FUNCTION "Gest Consensi 2ndCC" : VOID
TITLE =
VERSION : 0.1

BEGIN
NETWORK
TITLE =Condizioni di Sicurezza OK
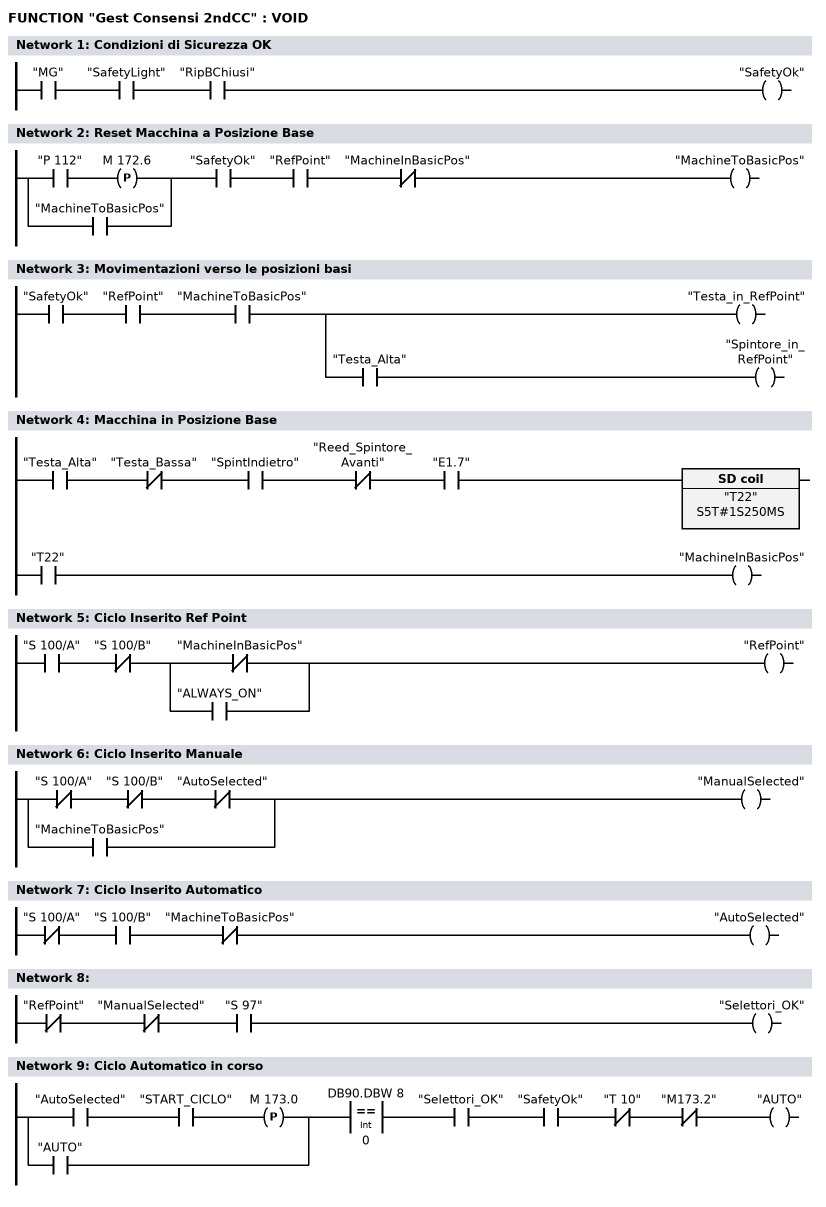
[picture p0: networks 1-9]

      U     "MG";
      U     "SafetyLight";
      U     "RipBChiusi";
      =     "SafetyOk";
NETWORK
TITLE =Reset Macchina a Posizione Base

      U(    ;
      U     "P 112";
      FP    M    172.6;
      O     "MachineToBasicPos";
      )     ;
      U     "SafetyOk";
      U     "RefPoint";
      UN    "MachineInBasicPos";
      =     "MachineToBasicPos";
NETWORK
TITLE =Movimentazioni verso le posizioni basi

      U     "SafetyOk";
      U     "RefPoint";
      U     "MachineToBasicPos";
      =     L      0.0;
      U     L      0.0;
      BLD   102;
      =     "Testa_in_RefPoint";
      U     L      0.0;
      U     "Testa_Alta";
      =     "Spintore_in_RefPoint";
NETWORK
TITLE =Macchina in Posizione Base

      U     "Testa_Alta";
      UN    "Testa_Bassa";
      U     "SpintIndietro";
      UN    "Reed_Spintore_Avanti";
      U     "E1.7";
      L     S5T#1S250MS;
      SE    "T22";
      NOP   0;
      NOP   0;
      NOP   0;
      U     "T22";
      =     "MachineInBasicPos";
NETWORK
TITLE =Ciclo Inserito Ref Point

      U     "S 100/A";
      UN    "S 100/B";
      U(    ;
      ON    "MachineInBasicPos";
      O     "ALWAYS_ON";
      )     ;
      =     "RefPoint";
NETWORK
TITLE =Ciclo Inserito Manuale

      UN    "S 100/A";
      UN    "S 100/B";
      UN    "AutoSelected";
      O     "MachineToBasicPos";
      =     "ManualSelected";
NETWORK
TITLE =Ciclo Inserito Automatico

      UN    "S 100/A";
      U     "S 100/B";
      UN    "MachineToBasicPos";
      =     "AutoSelected";
NETWORK
TITLE =

      UN    "RefPoint";
      UN    "ManualSelected";
      U     "S 97";
      =     "Selettori_OK";
NETWORK
TITLE =Ciclo Automatico in corso

      U(    ;
      U     "AutoSelected";
      U     "START_CICLO";
      FP    M    173.0;
      O     "AUTO";
      )     ;
      U(    ;
      L     DB90.DBW    8;
      L     0;
      ==I   ;
      )     ;
      U     "Selettori_OK";
      U     "SafetyOk";
      UN    "T 10";
      UN    "M173.2";
      =     "AUTO";
NETWORK
TITLE =Funzioni di toggle sul pulsante di start

      U(    ;
      U     "AUTO";
      UN    "START_CICLO";
      L     S5T#300MS;
      SE    "T40";
      NOP   0;
      NOP   0;
      NOP   0;
      U     "T40";
      )     ;
      S     "M173.1";
      U(    ;
      ON    "AUTO";
      ON    "AutoSelected";
      )     ;
      R     "M173.1";
      NOP   0;
NETWORK
TITLE =Impulso di Toggle
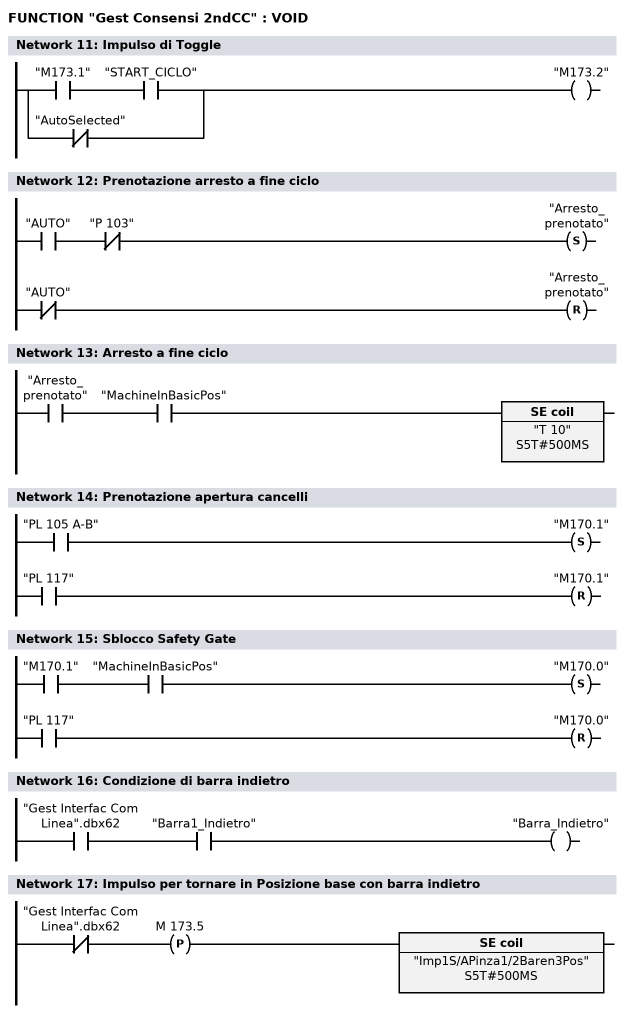
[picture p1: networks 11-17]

      U     "M173.1";
      U     "START_CICLO";
      ON    "AutoSelected";
      =     "M173.2";
NETWORK
TITLE =Prenotazione arresto a fine ciclo

      U     "AUTO";
      UN    "P 103";
      S     "Arresto_prenotato";
      UN    "AUTO";
      R     "Arresto_prenotato";
      NOP   0;
NETWORK
TITLE =Arresto a fine ciclo

      U     "Arresto_prenotato";
      U     "MachineInBasicPos";
      L     S5T#500MS;
      SV    "T 10";
      NOP   0;
      NOP   0;
      NOP   0;
      NOP   0;
NETWORK
TITLE =Prenotazione apertura cancelli

      U     "PL 105 A-B";
      S     "M170.1";
      U     "PL 117";
      R     "M170.1";
      NOP   0;
NETWORK
TITLE =Sblocco Safety Gate

      U     "M170.1";
      U     "MachineInBasicPos";
      S     "M170.0";
      U     "PL 117";
      R     "M170.0";
      NOP   0;
NETWORK
TITLE =Condizione di barra indietro

      U     "Gest Interfac Com Linea".dbx62;
      U     "Barra1_Indietro";
      =     "Barra_Indietro";
NETWORK
TITLE =Impulso per tornare in Posizione base con barra indietro

      UN    "Gest Interfac Com Linea".dbx62;
      FP    M    173.5;
      L     S5T#500MS;
      SV    "Imp1S/APinza1/2Baren3Pos";
      NOP   0;
      NOP   0;
      NOP   0;
      NOP   0;
END_FUNCTION

